PROGRAM MAIN
VAR
	IDENTControl_FB_Head1		: IDENTControl_SF;			(*Function block for channel 1*)
	IDENTControl_FB_Head2		: IDENTControl_SF;			(*Function block for channel 2*)

	Head1Data					: IDENTControl_UserData;	(*Data block for read/write data of channel 1*)
	Head2Data 					: IDENTControl_UserData;	(*Data block for read/write data of channel 2*)
		
	Head1SetRestart				: BOOL;						(*Trigger initialisation routine*)
	Head1InitFinish				: BOOL;						(*Initialisation routine finished*)
	Head1Quit					: BOOL;						(*Trigger Quit command to about Enhanced command*)
	Head1Read					: BOOL;						(*Trigger Read command*)
	Head1UserMemoryUID			: BOOL;						(*0 := access to User Memory; 1 := access to UID/Fixcode*)		
	Head1EPC 					: BOOL;						(*0 := configuration done by Head1UserMemoryUID active; 1 := access to UII/EPC Code (UHF only)*)
	Head1Busy					: BOOL;						(*0 = no command actiive; 1 = command active*)
	Head1Done					: BOOL;						(*0 = tag leave detection zone (Enhanced); 1 = tag access successfully executed*)
	Head1Finish 				: BOOL;						(*0 = command active; 1 = command finished*)		
	Head1Status					: BYTE;						(*Status value of the command response; error information*)
	Head1ReplyCounter			: BYTE;						(*Counter of the command responses; increment each new response*)
	Head1Error					: BOOL;						(*0 = no error state; 1 = error state active; check status value*)
	Head1SingleEnhanced			: BOOL;						(*0 := execute a Single (one-time) command; 1 := execute an Enhanced (permanent) command*)
	Head1NoDataCarrier			: BOOL;						(*0 = tag inside/enter detection zone; 1 = no tag or tag leave detection zone*)
	Head1Write					: BOOL;						(*Trigger Write command*)
	Head1TagType 				: WORD := 16#3939;			(*Configuration of TagType; default = 16#3939 = "99"*)
	Head1StartAddress 			: WORD := 16#0000;			(*Configuration of start address on User Memory for tag access*)
	Head1WordNum 				: INT := 4;					(*Number of accessed 4-Byte blocks*)
	Head1SpecialCommand			: BOOL;						(*Trigger Special (user defined) command*)
	
	Head2SetRestart				: BOOL;						(*Trigger initialisation routine*)
	Head2InitFinish				: BOOL;						(*Initialisation routine finished*)
	Head2Quit					: BOOL;						(*Trigger Quit command to about Enhanced command*)
	Head2Read					: BOOL;						(*Trigger Read command*)
	Head2UserMemoryUID			: BOOL;						(*0 := access to User Memory; 1 := access to UID/Fixcode*)
	Head2EPC 					: BOOL;						(*0 := configuration done by Head1UserMemoryUID active; 1 := access to UII/EPC Code (UHF only)*)
	Head2Busy					: BOOL;						(*0 = no command actiive; 1 = command active*)
	Head2Done					: BOOL;						(*0 = tag leave detection zone (Enhanced); 1 = tag access successfully executed*)
	Head2Finish 				: BOOL;						(*0 = command active; 1 = command finished*)	
	Head2Status					: BYTE;						(*Status value of the command response; error information*)
	Head2ReplyCounter			: BYTE;						(*Counter of the command responses; increment each new response*)
	Head2Error					: BOOL;						(*0 = no error state; 1 = error state active; check status value*)
	Head2SingleEnhanced			: BOOL;						(*0 := execute a Single (one-time) command; 1 := execute an Enhanced (permanent) command*)
	Head2NoDataCarrier			: BOOL;						(*0 = tag inside/enter detection zone; 1 = no tag or tag leave detection zone*)
	Head2Write					: BOOL;						(*Trigger Write command*)
	Head2TagType 				: WORD := 16#3939;			(*Configuration of TagType; default = 16#3939 = "99"*)
	Head2StartAddress 			: WORD := 16#0000;			(*Configuration of start address on User Memory for tag access*)
	Head2WordNum 				: INT := 4;					(*Number of accessed 4-Byte blocks*)
	Head2SpecialCommand			: BOOL;						(*Trigger Special (user defined) command*)
END_VAR

(*Call function block for channel 1*)
IDENTControl_FB_Head1(
	pADR_IN	:= ADR(BUS_INPUT[1]),						(* Pointer array input data *)
	cbSIZE_IN := SIZEOF(BUS_INPUT[1]),					(* Size array input data *)
	pADR_OUT := ADR(BUS_OUTPUT[1]),						(* Pointer array output data *)
	cbSIZE_OUT := SIZEOF(BUS_OUTPUT[1]),				(* Size array output data *)
	I_T_Timeout := T#5S, 								// Timeout to check command responses
	I_b_StartRead := Head1Read, 						// Trigger to start read command
	I_b_StartWrite := Head1Write, 						// Trigger to start write command
	I_b_StartSpecialCommand	:= Head1SpecialCommand, 	// Trigger to start special command (user defined command)
	I_b_UserMemory_UID := Head1UserMemoryUID, 			//0 := access to User Memory; 1 := access to UID/Fixcode
	I_b_EPC := Head1EPC,								//0 := configuration done by Head1UserMemoryUID active; 1 := access to UII/EPC Code (UHF only)
	I_b_SingleEnhanced := Head1SingleEnhanced , 		// 0 = Single command (one-time) ; 1 = Enhanced command (permanent)
	I_b_Quit := Head1Quit, 								// Trigger to start Quit command (abort Enhanced command)
	I_w_StartAddress := Head1StartAddress, 				// Startaddress of memory access 
	I_i_WordNumber := Head1WordNum,						// Number of blocks 
	I_w_TagType := Head1TagType, 						// TagType
	O_b_Done => Head1Done, 								//0 = tag leave detection zone (Enhanced); 1 = tag access successfully executed
	O_b_NoDataCarrier => Head1NoDatacarrier, 			//0 = tag inside/enter detection zone; 1 = no tag or tag leave detection zone
	O_b_Busy => Head1Busy, 								//0 = no command actiive; 1 = command active
	O_b_Finish => Head1Finish, 							//0 = command active; 1 = command finished
	O_b_Error => Head1Error, 							//0 = no error state; 1 = error state active; check status value
	O_B_Status => Head1Status, 							//Status value of the command response; error information
	O_B_ReplyCounter => Head1ReplyCounter,				//Counter of the command responses; increment each new response
	IO_b_SetRestart := Head1SetRestart, 				//Trigger initialisation routine
	IO_b_InitFinish := Head1Initfinish,					//Initialisation routine finished
	UserData := Head1Data								//Data block for read/write data
	);
	
(*Call function block for channel 2*)	
IDENTControl_FB_Head2(
	pADR_IN	:= ADR(BUS_INPUT[2]),						(* Pointer array input data *)
	cbSIZE_IN := SIZEOF(BUS_INPUT[2]),					(* Size array input data *)
	pADR_OUT := ADR(BUS_OUTPUT[2]),						(* Pointer array output data *)
	cbSIZE_OUT := SIZEOF(BUS_OUTPUT[2]),				(* Size array output data *)
	I_T_Timeout := T#5S, 								// Timeout to check command responses
	I_b_StartRead := Head2Read, 						// Trigger to start read command
	I_b_StartWrite := Head2Write, 						// Trigger to start write command
	I_b_StartSpecialCommand	:= Head2SpecialCommand, 	// Trigger to start special command (user defined command)
	I_b_UserMemory_UID := Head2UserMemoryUID, 			//0 := access to User Memory; 1 := access to UID/Fixcode
	I_b_EPC := Head2EPC,								//0 := configuration done by Head1UserMemoryUID active; 1 := access to UII/EPC Code (UHF only)
	I_b_SingleEnhanced := Head2SingleEnhanced , 		// 0 = Single command (one-time) ; 1 = Enhanced command (permanent)
	I_b_Quit := Head2Quit, 								// Trigger to start Quit command (abort Enhanced command)
	I_w_StartAddress := Head2StartAddress, 				// Startaddress of memory access 
	I_i_WordNumber := Head2WordNum, 					// Number of blocks 
	I_w_TagType := Head2TagType, 						// TagType
	O_b_Done => Head2Done, 								//0 = tag leave detection zone (Enhanced); 1 = tag access successfully executed
	O_b_NoDataCarrier => Head2NoDatacarrier, 			//0 = tag inside/enter detection zone; 1 = no tag or tag leave detection zone
	O_b_Busy => Head2Busy, 								//0 = no command actiive; 1 = command active
	O_b_Finish => Head2Finish, 							//0 = command active; 1 = command finished
	O_b_Error => Head2Error, 							//0 = no error state; 1 = error state active; check status value
	O_B_Status => Head2Status, 							//Status value of the command response; error information
	O_B_ReplyCounter => Head2ReplyCounter,				//Counter of the command responses; increment each new response
	IO_b_SetRestart := Head2SetRestart, 				//Trigger initialisation routine
	IO_b_InitFinish := Head2Initfinish,					//Initialisation routine finished
	UserData := Head2Data								//Data block for read/write data
	);
	
	
IF Head1Read THEN Head1Read := FALSE; END_IF;
IF Head1Write THEN Head1Write := FALSE; END_IF;
IF Head1Quit THEN Head1Quit := FALSE; END_IF;
IF Head1SpecialCommand THEN Head1SpecialCommand := FALSE; END_IF;
IF Head2Read THEN Head2Read := FALSE; END_IF;
IF Head2Write THEN Head2Write := FALSE; END_IF;
IF Head2Quit THEN Head2Quit := FALSE; END_IF;
IF Head2SpecialCommand THEN Head2SpecialCommand := FALSE; END_IF;

END_PROGRAM
